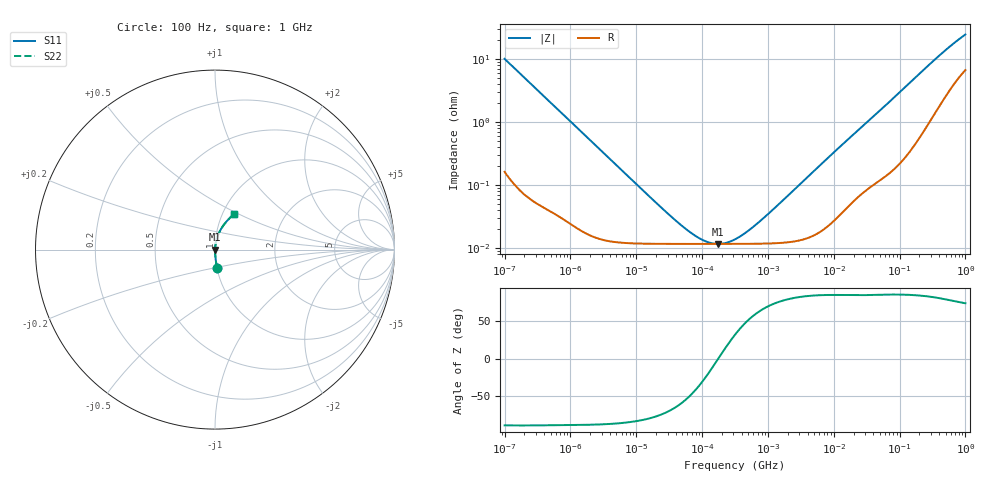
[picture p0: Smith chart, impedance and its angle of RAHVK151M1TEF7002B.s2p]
! RAHVK151M1TEF7002B  S-PARAMETER MODEL  (AEC-Q200 qualified)
! Model Generated by ELNA Corporation (http://www.ty-top.com)
! Version 1.0
! ELNA Control No. 240315
! Copyright (c) 2024 ELNA CO.,LTD. All Rights Reserved.
! Products Name : CONDUCTIVE POLYMER HYBRID ALUMINUM ELECTROLYTIC CAPACITORS
! Characteristics :
!  Capacitance  :  150uF  ,  Rated voltage  :  25V
!  Operating Temp. Range  :  -55 to +125 degC  ,  Endurance  :  6000hr at 125 degC
!  Dimension D  :  8mm  ,  Dimension L  :  8.7mm
! Frequency Range : 100Hz - 1GHz
! External Node Assignments :
!  1  o---| |---o  2
# MHz S RI R 50
!Freq[MHz].  S11 Real  S11 Imag  S21 Real  S21 Imag  S12 Real  S12 Imag  S22 Real  S22 Imag
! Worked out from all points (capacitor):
!   401 points, 100 Hz to 1 GHz, reference 50 ohm
!   read as one part in series: C = 156 uF near 108 Hz
!   lowest |Z| = 11.7 mohm at 172.8 kHz (marker M1)
!   series resonance near 175.9 kHz, so ESL is about 5.2 nH
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0.0001  0.0119 -0.1006  0.9881 0.1006  0.9881 0.1006  0.0119 -0.1006
0.000113  0.00945 -0.0894  0.9906 0.0894  0.9906 0.0894  0.00945 -0.0894
0.000309  0.0016 -0.033  0.9984 0.033  0.9984 0.033  0.0016 -0.033
0.001488  0.000236 -0.00698  0.9998 0.00698  0.9998 0.00698  0.000236 -0.00698
0.022131  0.000118 -0.000464  0.9999 0.000464  0.9999 0.000464  0.000118 -0.000464
0.045709  0.000117 -0.000213  0.9999 0.000213  0.9999 0.000213  0.000117 -0.000213
0.077179  0.000117 -0.000109  0.9999 0.000109  0.9999 0.000109  0.000117 -0.000109
0.098288  0.000117 -7.3e-05  0.9999 7.3e-05  0.9999 7.3e-05  0.000117 -7.3e-05
0.120226  0.000117 -4.62e-05  0.9999 4.62e-05  0.9999 4.62e-05  0.000117 -4.62e-05
0.172783  0.000117 -2.1e-06  0.9999 2.1e-06  0.9999 2.1e-06  0.000117 -2.1e-06
0.229087  0.000117 3.17e-05  0.9999 -3.17e-05  0.9999 -3.17e-05  0.000117 3.17e-05
0.316228  0.000117 7.37e-05  0.9999 -7.37e-05  0.9999 -7.37e-05  0.000117 7.37e-05
0.473151  0.000118 0.000138  0.9999 -0.000138  0.9999 -0.000138  0.000118 0.000138
0.767361  0.000118 0.000245  0.9999 -0.000245  0.9999 -0.000245  0.000118 0.000245
1.462177  0.000121 0.000486  0.9999 -0.000486  0.9999 -0.000486  0.000121 0.000486
4.704354  0.000158 0.00158  0.9998 -0.00158  0.9998 -0.00158  0.000158 0.00158
12.8825  0.000369 0.00423  0.9996 -0.00423  0.9996 -0.00423  0.000369 0.00423
69.9842  0.00199 0.021  0.998 -0.021  0.998 -0.021  0.00199 0.021
176.8072  0.00731 0.0515  0.9927 -0.0515  0.9927 -0.0515  0.00731 0.0515
395.8221  0.029 0.1069  0.971 -0.1069  0.971 -0.1069  0.029 0.1069
668.3439  0.0654 0.158  0.9346 -0.158  0.9346 -0.158  0.0654 0.158
1000  0.108 0.1997  0.892 -0.1997  0.892 -0.1997  0.108 0.1997
